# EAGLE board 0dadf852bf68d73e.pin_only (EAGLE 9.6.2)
REV: B

Size 80.77 x 53.34 mm. Coordinates in mm from the lower left corner, seen from the top.
Outline: 0,0 80.77,0 80.77,53.34 0,53.34 0,0
Copper layers (1*16): Top 0.035mm / dielectric 1.5mm / Bottom 0.035mm
Design rules "adafruit 8-8": minimum track width 6mil, minimum drill 15.5mil, track to track 8mil, track to pad 8mil, pad to pad 8mil, via to via 8mil, smd to smd 8mil, copper to edge 10mil, drill to drill 8mil, minimum pad ring 10mil, minimum via ring 8mil, stop-mask expansion 2mil, vias tented up to drill 20mil, thermal gap 10mil

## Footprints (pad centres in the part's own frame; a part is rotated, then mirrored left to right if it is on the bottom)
0805-NO = smd 1.24 x 1.5: 1 -0.95,0; 2 0.95,0
6MMX6MM_TACTILE_SMT = smd 2 x 1.2: A -3.5,-2.25; A' 3.5,-2.25; B -3.5,2.25; B' 3.5,2.25
FIDUCIAL_1MM = smd 1 x 1: 1 0,0
SSOP28 = smd 0.4 x 1.5: 1 -4.225,-3.625; 2 -3.575,-3.625; 3 -2.925,-3.625; 4 -2.275,-3.625; 5 -1.625,-3.625; 6 -0.975,-3.625; 7 -0.325,-3.625; 8 0.325,-3.625; 9 0.975,-3.625; 10 1.625,-3.625; 11 2.275,-3.625; 12 2.925,-3.625; 13 3.575,-3.625; 14 4.225,-3.625; 15 4.225,3.625; 16 3.575,3.625; 17 2.925,3.625; 18 2.275,3.625; 19 1.625,3.625; 20 0.975,3.625; 21 0.325,3.625; 22 -0.325,3.625; 23 -0.975,3.625; 24 -1.625,3.625; 25 -2.275,3.625; 26 -2.925,3.625; 27 -3.575,3.625; 28 -4.225,3.625
SOLDERJUMPER_2WAY_OPEN_NOPASTE = smd 1.168 x 1.6: 1 -1.397,0; 2 0,0; 3 1.397,0
SOLDERJUMPER_ARROW_NOPASTE = smd 0.762 x 1.524: 1 -1.016,0; 2 1.016,0
RTRIM3314J = smd 1.3 x 2: 1 1.2,-2; 3 -1.2,-2 | smd 2 x 2: 2 0,1.9
ARDUINOR3-NOTEXT-NOIOREF = drill 1 pad 1.676 octagon: 3V 35.56,2.54; 5V 38.1,2.54; A0 50.8,2.54; A1 53.34,2.54; A2 55.88,2.54; A3 58.42,2.54; A4 60.96,2.54; A5 63.5,2.54; AREF 23.876,50.8; D0 63.5,50.8; D1 60.96,50.8; D2 58.42,50.8; D3 55.88,50.8; D4 53.34,50.8; D5 50.8,50.8; D6 48.26,50.8; D7 45.72,50.8; D8 41.656,50.8; D9 39.116,50.8; D10 36.576,50.8; D11 34.036,50.8; D12 31.496,50.8; D13 28.956,50.8; GND 26.416,50.8; GND1 43.18,2.54; GND2 40.64,2.54; RESET 33.02,2.54; SCL 18.796,50.8; SDA 21.336,50.8; VIN 45.72,2.54
LCD1602-RGB = drill 1 pad 1.778: 1 -32,15.5; 2 -29.46,15.5; 3 -26.92,15.5; 4 -24.38,15.5; 5 -21.84,15.5; 6 -19.3,15.5; 7 -16.76,15.5; 8 -14.22,15.5; 9 -11.68,15.5; 10 -9.14,15.5; 11 -6.6,15.5; 12 -4.06,15.5; 13 -1.52,15.5; 14 1.02,15.5; 15 3.56,15.5; 16 6.1,15.5; 17 8.64,15.5; 18 11.18,15.5 | hole 2.8: -37.5,-15.5; -37.5,15.5; 37.5,15.5; 37.5,-15.5

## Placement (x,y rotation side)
BLUE  220  [0805-NO]  56.9,8.76 270 top
DOWN  6mm  [6MMX6MM_TACTILE_SMT]  11.43,3.56 0 top
E$1  [PCBFEAT-REV-040]  78.61,51.82 0 top
FID1  FIDUCIAL_1MM  [FIDUCIAL_1MM]  2.79,20.95 0 top
FID2  FIDUCIAL_1MM  [FIDUCIAL_1MM]  5.84,48.64 0 top
FID3  FIDUCIAL_1MM  [FIDUCIAL_1MM]  77.98,21.21 0 top
GRN  330  [0805-NO]  54.86,8.76 90 top
IC1  MCP23017SS  [SSOP28]  46.48,9.27 180 top
LEFT  6mm  [6MMX6MM_TACTILE_SMT]  3.81,6.99 270 top
PLABEL1  [PLABEL1]  0.89,51.05 0 top
PLABEL2  [PLABEL2]  65.91,51.05 0 top
PLABEL3  [PLABEL3]  63.5,8.13 0 top
PLABEL4  [PLABEL4]  35.56,4.32 0 top
PLABEL5  [PLABEL5]  34.04,8.51 90 top
PLABEL6  [PLABEL6]  36.96,8.51 90 top
PLABEL7  [PLABEL7]  59.18,5.46 90 top
PLABEL8  [PLABEL8]  65.28,5.33 90 top
PLABEL9  [PLABEL9]  16,12.57 0 top
PLABEL10  [PLABEL10]  0.25,0.25 0 top
PLABEL11  [PLABEL11]  2.03,11.81 0 top
PLABEL12  [PLABEL12]  16.38,0.64 0 top
PLABEL13  [PLABEL13]  24.64,5.08 0 top
PLABEL14  [PLABEL14]  66.04,2.29 0 top
PLABEL15  [PLABEL15]  79.38,6.99 90 top
R1  4.7K  [0805-NO]  40.01,8.13 270 top
R2  4.7K  [0805-NO]  40.01,12.32 90 top
RED  220  [0805-NO]  52.96,8.76 270 top
RESET  6mm  [6MMX6MM_TACTILE_SMT]  75.44,3.3 0 top
RIGHT  6mm  [6MMX6MM_TACTILE_SMT]  19.05,6.99 90 top
SELECT  6mm  [6MMX6MM_TACTILE_SMT]  27.94,10.16 0 top
SJ1  [SOLDERJUMPER_2WAY_OPEN_NOPASTE]  35.56,6.22 180 top
SJ2  [SOLDERJUMPER_ARROW_NOPASTE]  63.5,5.46 90 top
SJ3  [SOLDERJUMPER_ARROW_NOPASTE]  60.96,5.46 270 top
TM1  10K  [RTRIM3314J]  75.44,10.41 0 top
U1  ARDUINOR3-NOIOREF-NOTEXT  [ARDUINOR3-NOTEXT-NOIOREF]  0,0 0 top
U$1  HD44780LCD_RGBLONGPINS  [LCD1602-RGB]  40.39,32.51 0 top
U$4  [ADAFRUIT_3.5MM]  65.91,9.91 0 top
UP  6mm  [6MMX6MM_TACTILE_SMT]  11.43,10.16 0 top

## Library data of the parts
BLUE E$1 GRN R1 R2 RED SJ1 U$4 = microbuilder
DOWN LEFT RESET RIGHT SELECT UP = adafruit_electromech
FID1-FID3 SJ2 SJ3 = microbuilder; BOM: EXCLUDE
IC1 U1 U$1 = adafruit
PLABEL1-PLABEL15 = pinguin
TM1 = adafruit_electromech; SPICEMODEL: X; SPICEPREFIXL: POT

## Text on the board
Pinguin_tBackup: i2c 16x2 RGB | LCD shield | Left | Up | 3V | 5V | adafruit! | Contrast | Contrast | Select | SDA | SCL | Vio | Reset | Down | Right

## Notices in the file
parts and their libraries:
microbuilder: This work is placed in the public domain, and may be freely used for commercial and non-commercial work with the following conditions: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
